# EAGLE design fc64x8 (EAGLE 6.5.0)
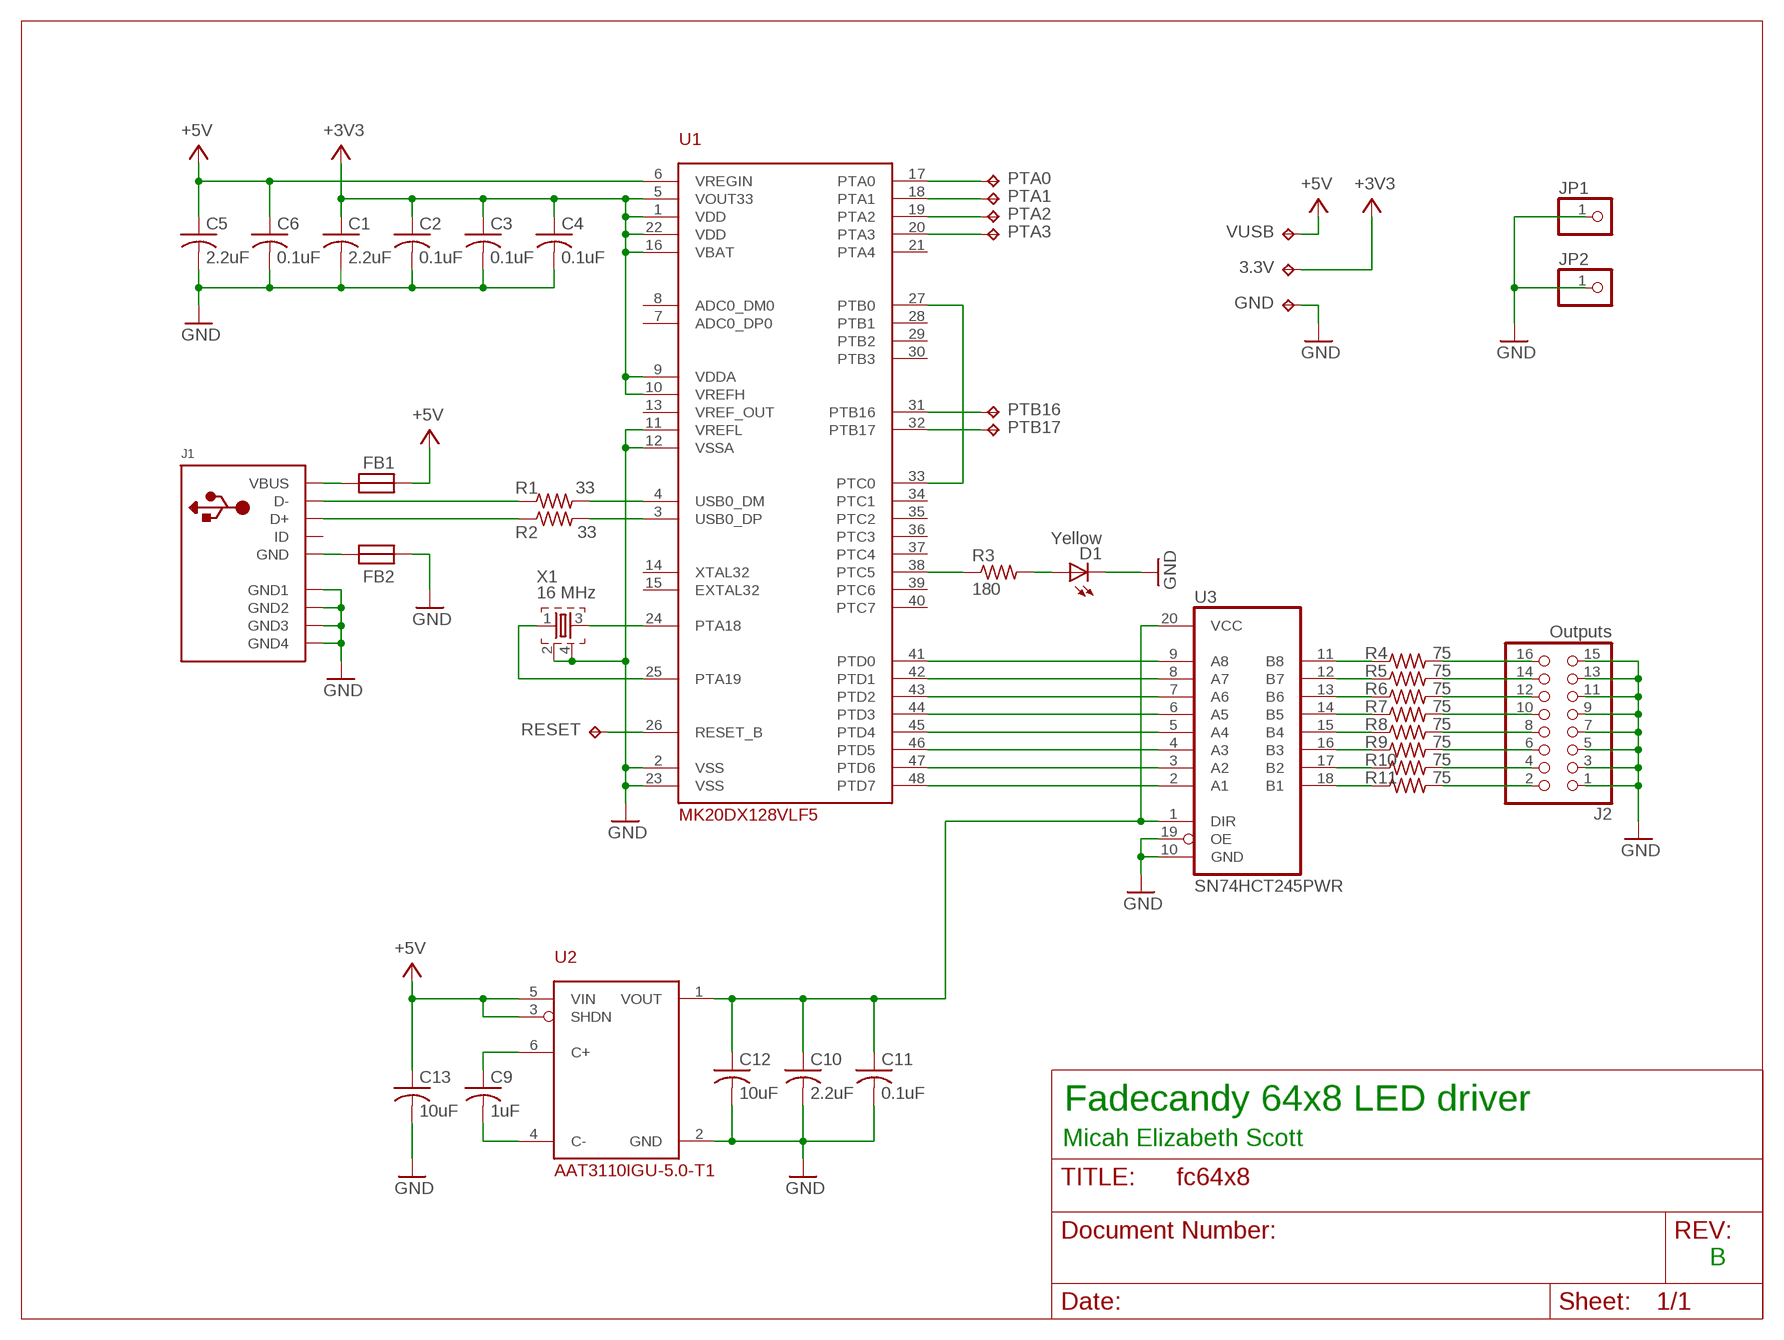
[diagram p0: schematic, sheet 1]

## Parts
3.3V  TPTP18SQ  [TP18SQ]
C1  2.2uF  C-US0805/NO-OUTLINE  [0805]
C2  0.1uF  C-US0805/NO-OUTLINE  [0805]
C3  0.1uF  C-US0805/NO-OUTLINE  [0805]
C4  0.1uF  C-US0805/NO-OUTLINE  [0805]
C5  2.2uF  C-US0805/NO-OUTLINE  [0805]
C6  0.1uF  C-US0805/NO-OUTLINE  [0805]
C9  1uF  C-US0805/NO-OUTLINE  [0805]
C10  2.2uF  C-US0805/NO-OUTLINE  [0805]
C11  0.1uF  C-US0805/NO-OUTLINE  [0805]
C12  10uF  C-US0805/NO-OUTLINE  [0805]
C13  10uF  C-US0805/NO-OUTLINE  [0805]
D1  Yellow  LEDCHIP-LED0805  [CHIP-LED0805]
FB1  FB0805/NO-OUTLINE  [0805]
FB2  FB0805/NO-OUTLINE  [0805]
GND  TPTP18SQ  [TP18SQ]
J1  USBMINIB  [USB-MINIB]
J2  Outputs  PINHD-2X8  [2X08]
JP1  PINHD-1X1  [1X01]
JP2  PINHD-1X1  [1X01]
PTA0  TPTP18SQ  [TP18SQ]
PTA1  TPTP18SQ  [TP18SQ]
PTA2  TPTP18SQ  [TP18SQ]
PTA3  TPTP18SQ  [TP18SQ]
PTB16  TPTP18SQ  [TP18SQ]
PTB17  TPTP18SQ  [TP18SQ]
R1  33  R-US_0805/NO-OUTLINE  [0805]
R2  33  R-US_0805/NO-OUTLINE  [0805]
R3  180  R-US_0805/NO-OUTLINE  [0805]
R4  75  R-US_0805/NO-OUTLINE  [0805]
R5  75  R-US_0805/NO-OUTLINE  [0805]
R6  75  R-US_0805/NO-OUTLINE  [0805]
R7  75  R-US_0805/NO-OUTLINE  [0805]
R8  75  R-US_0805/NO-OUTLINE  [0805]
R9  75  R-US_0805/NO-OUTLINE  [0805]
R10  75  R-US_0805/NO-OUTLINE  [0805]
R11  75  R-US_0805/NO-OUTLINE  [0805]
RESET  TPTP18SQ  [TP18SQ]
U1  MK20DX128VLF5  [LQFP48]
U2  AAT3110IGU-5.0-T1  AAT3110  [SOT23-6L]
U3  SN74HCT245PWR  74245PW  [TSSOP20]
VUSB  TPTP18SQ  [TP18SQ]
X1  16 MHz  TSX-32250  [TSX-3225]

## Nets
+3V3: 3.3V.TP C1.1 C2.1 C3.1 C4.1 U1.1(VDD) U1.5(VOUT33) U1.9(VDDA) U1.10(VREFH) U1.16(VBAT) U1.22(VDD)
+5V: C5.1 C6.1 C13.1 FB1.2 U1.6(VREGIN) U2.3(SHDN) U2.5(VIN) VUSB.TP
GND: C1.2 C2.2 C3.2 C4.2 C5.2 C6.2 C10.2 C11.2 C12.2 C13.2 D1.C FB2.2 GND.TP J1.GND1 J1.GND2 J1.GND3 J1.GND4 J2.1 J2.3 J2.5 J2.7 J2.9 J2.11 J2.13 J2.15 JP1.1 JP2.1 U1.2(VSS) U1.11(VREFL) U1.12(VSSA) U1.23(VSS) U2.2(GND) U3.10(GND) U3.19(OE) X1.2 X1.4
N$1: R3.1 U1.38(PTC5)
N$2: U1.24(PTA18) X1.3
N$3: D1.A R3.2
N$4: U1.25(PTA19) X1.1
N$5: FB1.1 J1.VBUS
N$6: U1.27(PTB0) U1.33(PTC0)
N$7: FB2.1 J1.GND
N$8: U1.41(PTD0) U3.9(A8)
N$9: J1.D- R1.1
N$10: J1.D+ R2.1
N$11: R1.2 U1.4(USB0_DM)
N$12: R2.2 U1.3(USB0_DP)
N$13: U1.42(PTD1) U3.8(A7)
N$14: U1.43(PTD2) U3.7(A6)
N$15: U1.44(PTD3) U3.6(A5)
N$16: U1.45(PTD4) U3.5(A4)
N$17: U1.46(PTD5) U3.4(A3)
N$18: U1.47(PTD6) U3.3(A2)
N$19: U1.48(PTD7) U3.2(A1)
N$20: R4.1 U3.11(B8)
N$21: C9.1 U2.6(C+)
N$22: C9.2 U2.4(C-)
N$23: R5.1 U3.12(B7)
N$24: R6.1 U3.13(B6)
N$25: R7.1 U3.14(B5)
N$26: R8.1 U3.15(B4)
N$27: C10.1 C11.1 C12.1 U2.1(VOUT) U3.1(DIR) U3.20(VCC)
N$28: R9.1 U3.16(B3)
N$29: R10.1 U3.17(B2)
N$30: R11.1 U3.18(B1)
N$31: J2.16 R4.2
N$32: J2.14 R5.2
N$33: J2.12 R6.2
N$34: J2.10 R7.2
N$35: J2.8 R8.2
N$36: J2.6 R9.2
N$37: J2.4 R10.2
N$38: J2.2 R11.2
N$39: RESET.TP U1.26(RESET_B)
N$40: PTA0.TP U1.17(PTA0)
N$41: PTA1.TP U1.18(PTA1)
N$42: PTA2.TP U1.19(PTA2)
N$43: PTA3.TP U1.20(PTA3)
N$45: PTB16.TP U1.31(PTB16)
N$46: PTB17.TP U1.32(PTB17)
Unconnected: J1.ID U1.7(ADC0_DP0) U1.8(ADC0_DM0) U1.13(VREF_OUT) U1.14(XTAL32) U1.15(EXTAL32) U1.21(PTA4) U1.28(PTB1) U1.29(PTB2) U1.30(PTB3) U1.34(PTC1) U1.35(PTC2) U1.36(PTC3) U1.37(PTC4) U1.39(PTC6) U1.40(PTC7)

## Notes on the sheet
- Fadecandy 64x8 LED driver
- Micah Elizabeth Scott
- B

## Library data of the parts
3.3V GND PTA0 PTA1-PTA3 PTB16 PTB17 RESET VUSB = testpad:TP: Test pad
C1-C6 C9-C13 = scanlime:C-US: CAPACITOR, American symbol
D1 = adafruit:LED: LED
FB1 FB2 = scanlime:FB
J1 = scanlime:USB: USB Connectors USBMINIB - Surface Mount Female Mini-B USB Connector 4UConnector: 06564 By microbuilder.eu Thru-hole RA Female Mini-B USB Connector 4UConnector: 18732 By ladyada.net
J2 = pinhead:PINHD-2X8: PIN HEADER
JP1 JP2 = pinhead:PINHD-1X1: PIN HEADER
R1-R11 = scanlime:R-US_: RESISTOR, American symbol
U1 = scanlime:MK20DX128VLF5: ARM Cortex-M4 microcontroller with USB. Freescale K20 series 50 MHz 16 K RAM 128 K Flash Lower pincount equivalent to Teensy 3.0 2013 Price: $2.66 qty 100 Digi-Key: MK20DX128VLF50-ND
U2 = scanlime:AAT3110: Switched capacitor boost converter
U3 = scanlime:74*245: Octal BUS TRANSCEIVER, 3-state
X1 = scanlime:TSX-3225: MHz RANGE CRYSTAL UNIT Source: Epson Toyocom

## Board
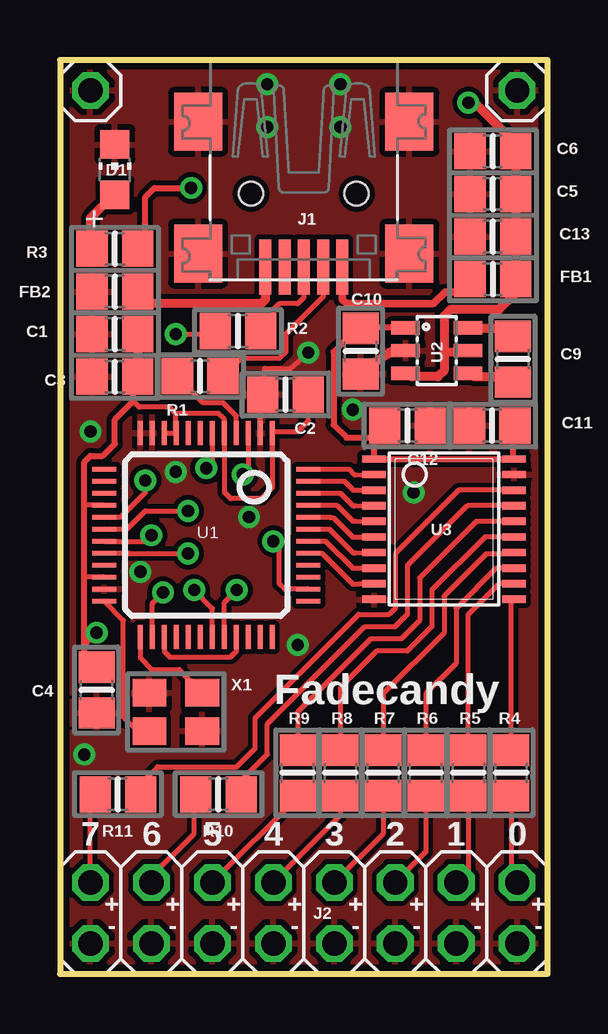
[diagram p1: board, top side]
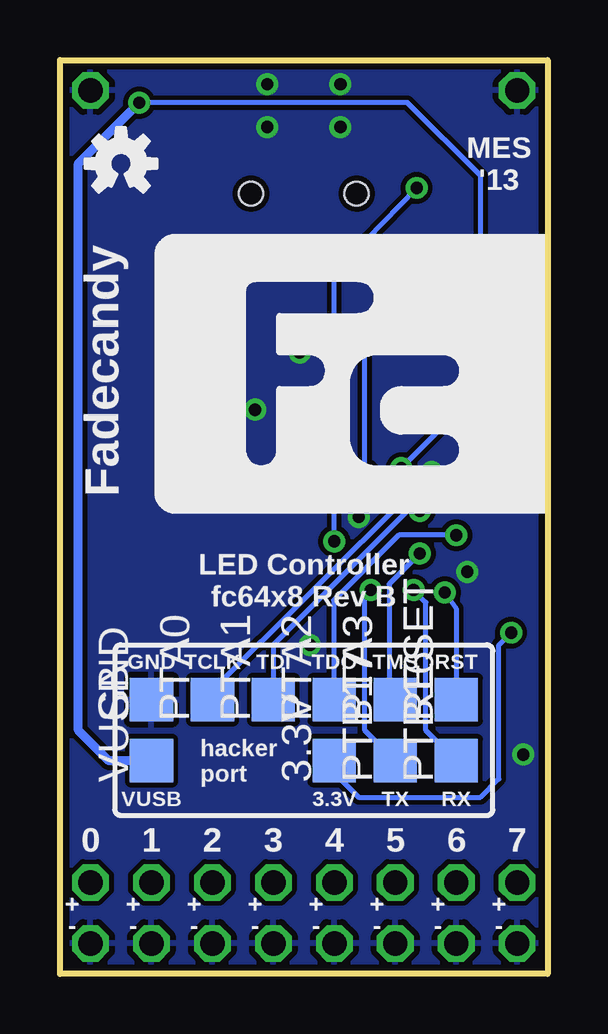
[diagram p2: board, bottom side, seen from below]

Size 20.32 x 38.1 mm. Coordinates in mm from the lower left corner, seen from the top.
Outline: 0,0 20.32,0 20.32,38.1 0,38.1 0,0
Copper layers (1*16): Top 0.035mm / dielectric 1.5mm / Bottom 0.035mm
Design rules "adafruit": minimum track width 8mil, minimum drill 15.5mil, track to track 8mil, track to pad 8mil, pad to pad 8mil, via to via 8mil, smd to smd 8mil, copper to edge 10mil, drill to drill 8mil, minimum pad ring 10mil, minimum via ring 8mil, stop-mask expansion 4mil, vias tented up to drill 20mil, thermal gap 10mil

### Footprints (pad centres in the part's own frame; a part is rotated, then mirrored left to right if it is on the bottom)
TP18SQ = smd 1.8 x 1.8: TP 0,0
0805 = smd 1.3 x 1.5: 1 -0.95,0; 2 0.95,0
CHIP-LED0805 = smd 1.2 x 1.2: A 0,-1.05; C 0,1.05
USB-MINIB = smd 0.5 x 2.308: D+ 0,4.064; D- -0.8,4.064; GND 1.6,4.064; ID 0.8,4.064; VBUS -1.6,4.064 | smd 2 x 2.4: GND1 -4.4,-2; GND2 -4.4,3.5; GND3 4.4,3.5; GND4 4.4,-2 | hole 1: -2.2,1; 2.2,1
2X08 = drill 1.016 octagon: 1 -8.89,-1.27; 2 -8.89,1.27; 3 -6.35,-1.27; 4 -6.35,1.27; 5 -3.81,-1.27; 6 -3.81,1.27; 7 -1.27,-1.27; 8 -1.27,1.27; 9 1.27,-1.27; 10 1.27,1.27; 11 3.81,-1.27; 12 3.81,1.27; 13 6.35,-1.27; 14 6.35,1.27; 15 8.89,-1.27; 16 8.89,1.27
1X01 = drill 1.016 octagon: 1 0,0
LQFP48 = smd 0.203 x 1: 1 -2.75,-4.25; 2 -2.25,-4.25; 3 -1.75,-4.25; 4 -1.25,-4.25; 5 -0.75,-4.25; 6 -0.25,-4.25; 7 0.25,-4.25; 8 0.75,-4.25; 9 1.25,-4.25; 10 1.75,-4.25; 11 2.25,-4.25; 12 2.75,-4.25; 25 2.75,4.25; 26 2.25,4.25; 27 1.75,4.25; 28 1.25,4.25; 29 0.75,4.25; 30 0.25,4.25; 31 -0.25,4.25; 32 -0.75,4.25; 33 -1.25,4.25; 34 -1.75,4.25; 35 -2.25,4.25; 36 -2.75,4.25 | smd 1 x 0.203: 13 4.25,-2.75; 14 4.25,-2.25; 15 4.25,-1.75; 16 4.25,-1.25; 17 4.25,-0.75; 18 4.25,-0.25; 19 4.25,0.25; 20 4.25,0.75; 21 4.25,1.25; 22 4.25,1.75; 23 4.25,2.25; 24 4.25,2.75; 37 -4.25,2.75; 38 -4.25,2.25; 39 -4.25,1.75; 40 -4.25,1.25; 41 -4.25,0.75; 42 -4.25,0.25; 43 -4.25,-0.25; 44 -4.25,-0.75; 45 -4.25,-1.25; 46 -4.25,-1.75; 47 -4.25,-2.25; 48 -4.25,-2.75
SOT23-6L = smd 0.55 x 1.2: 1 -0.95,-1.3; 2 0,-1.3; 3 0.95,-1.3; 4 0.95,1.3; 5 0,1.3; 6 -0.95,1.3
TSSOP20 = smd 0.305 x 0.991: 1 -2.925,-2.918; 2 -2.275,-2.918; 3 -1.625,-2.918; 4 -0.975,-2.918; 5 -0.325,-2.918; 6 0.325,-2.918; 7 0.975,-2.918; 8 1.625,-2.918; 9 2.275,-2.918; 10 2.925,-2.918; 11 2.925,2.918; 12 2.275,2.918; 13 1.625,2.918; 14 0.975,2.918; 15 0.325,2.918; 16 -0.325,2.918; 17 -0.975,2.918; 18 -1.625,2.918; 19 -2.275,2.918; 20 -2.925,2.918
TSX-3225 = smd 1.4 x 1.15: 1 -1.1,-0.8; 2 1.1,-0.8; 3 1.1,0.8; 4 -1.1,0.8

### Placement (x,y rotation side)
3.3V  8.89,8.89 90 bottom
C1  2.29,26.67 180 top
C2  9.4,24.16 180 top
C3  2.29,24.89 180 top
C4  1.52,11.84 270 top
C5  18.03,32.51 180 top
C6  18.03,34.29 180 top
C9  18.87,25.63 270 top
C10  12.52,25.96 270 top
C11  18.01,22.86 180 top
C12  14.48,22.86 0 top
C13  18.03,30.73 180 top
D1  2.29,33.53 0 top
FB1  18.03,28.96 0 top
FB2  2.29,28.45 180 top
GND  16.51,11.43 90 bottom
J1  10.16,33.53 180 top
J2  10.16,2.54 0 top
JP1  1.27,36.83 0 top
JP2  19.05,36.83 0 top
PTA0  13.97,11.43 90 bottom
PTA1  11.43,11.43 90 bottom
PTA2  8.89,11.43 90 bottom
PTA3  6.35,11.43 90 bottom
PTB16  3.81,8.89 90 bottom
PTB17  6.35,8.89 90 bottom
R1  5.84,24.92 180 top
R2  7.42,26.8 180 top
R3  2.29,30.23 180 top
R4  18.8,8.38 270 top
R5  17.02,8.38 270 top
R6  15.24,8.38 270 top
R7  13.46,8.38 270 top
R8  11.68,8.38 270 top
R9  9.91,8.38 270 top
R10  6.6,7.49 180 top
R11  2.41,7.49 180 top
RESET  3.81,11.43 90 bottom
U1  6.1,18.29 180 top
U2  15.7,25.98 270 top
U3  16,18.54 270 top
U$1  [OSHW-LOGO-S]  17.78,33.78 0 bottom
VUSB  16.51,8.89 90 bottom
X1  4.83,10.92 180 top

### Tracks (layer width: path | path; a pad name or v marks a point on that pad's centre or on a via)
+3V3  (via drill 0.51)
  Top 0.203: 1.02,16.51 1.04,16.54 U1.22 | 1.04,19.54 1.02,19.56 U1.16 | 1.02,13.46 1.02,13.72 v1.52,14.22 | U1.10 U1.9 | 1.02,12.95 C4.1 | U1.1 8.91,22.61 9.91,22.61 10.35,23.05 C2.1 | U1.9 4.83,22.56 4.83,23.37 | U1.1 8.89,22.58 | U1.9 4.83,22.52 | 8.85,21.8 U1.1 | 4.83,23.37 4.57,23.62 3.3,23.62 3.05,23.88 | U1.1 8.85,20.28 8.38,19.81 7.11,19.81 6.86,20.07 6.86,22.53 U1.5 6.85,23.13 6.6,23.37 4.83,23.37
  Top 0.254: 1.02,12.95 1.02,13.46 1.02,16.51 1.02,19.56 1.02,21.34 1.27,21.59 1.78,21.59 2.29,22.1 2.29,23.11 3.05,23.88 3.05,24.7 C3.1
  Top 0.381: C1.1 C3.1
  Bottom 0.203: 3.3V.TP 8.89,8.38 7.87,7.37 2.79,7.37 2.03,8.13 2.03,13.72 v1.52,14.22
+5V  (via drill 0.51)
  Top 0.203: 18.8,34.8 18.8,34.48 C6.1 | U1.6 6.35,21.33 v6.1,21.08
  Top 0.381: C6.1 C5.1 C13.1 FB1.2 18.98,28.38 18.29,27.69 16.26,27.69 16,27.43 16,25.91 | 16,25.91 16,25.15 15.75,24.89 14.67,24.89 U2.3 | U2.5 16.03,25.88 16,25.91 | v17.02,36.32 17.27,36.32 18.8,34.8
  Bottom 0.203: v6.1,21.08 2.79,24.38 2.79,33.27 5.84,36.32 v17.02,36.32
  Bottom 0.381: VUSB.TP 18.29,8.89 19.56,10.16 19.56,33.78 v17.02,36.32
GND  (via drill 0.51)
  Top 0.203: U1.2 8.35,24.03 C2.2 8.52,25.03 8.53,25.22 | 9.58,25.22 v10.34,25.91
  Top 0.254: 8.53,25.22 9.58,25.22
  Top 0.381: U2.2 13.89,25.98 13.01,25.43 12.86,25.3 C10.2
  other vias: 1.02,9.14 14.73,20.07 7.87,19.05 1.27,22.61 3.35,16.76 4.83,20.93 12.19,23.52 8.64,35.31 11.68,35.31 9.91,13.72 8.64,37.08 11.68,37.08
  pour Bottom: 0,38.1 20.32,38.1 20.32,0 0,0
  pour Top: 0,38.1 20.32,38.1 20.32,0 0,0
N$1  (via drill 0.51)
  Top 0.203: 3.56,30.55 R3.1 | U1.38 9.36,16.04 9.14,16.26 9.14,17.78 v8.89,18.03
  Top 0.254: 3.56,30.55 3.56,32.38 3.94,32.77 v5.46,32.77
  Bottom 0.203: v8.89,18.03 8.89,29.21 v5.46,32.77
N$2
  Top 0.203: X1.3 3.21,10.12 2.64,10.69 2.64,14.74 U1.24
N$3
  Top 0.381: D1.A 2.25,32.48 1.27,31.5 1.27,30.29 R3.2
N$4
  Top 0.203: U1.25 3.35,13.16 3.81,12.7 4.95,12.7 X1.1
N$5
  Top 0.305: J1.VBUS 11.76,28.12 11.94,27.94 15.56,27.94 16.05,28.42 16.94,28.42
  Top 0.381: 16.94,28.42 FB1.1
N$6
  Top 0.203: U1.27 4.35,13.43 4.57,13.21 7.11,13.21 7.35,13.44 U1.33
N$7
  Top 0.381: J1.GND 8.56,28.12 8.38,27.94 3.49,27.94 FB2.1
N$8
  Top 0.203: 12.45,16.26 U3.9 12.31,16.26 12.19,16.26 10.91,17.54 U1.41
N$9
  Top 0.203: J1.D- 10.96,28.23 9.4,26.67 9.4,25.91 9.14,25.65 7.53,25.65 R1.1
N$10
  Top 0.203: J1.D+ 10.16,28.19 9.91,27.94 9.14,27.94 8.89,27.69 8.89,27.32 R2.1
N$11
  Top 0.203: U1.4 7.35,23.26 6.81,23.8 5.96,23.8 R1.2
N$12  (via drill 0.51)
  Top 0.203: U1.3 7.85,21.05 v7.62,20.83 | v4.83,26.67 6.39,26.67 R2.2
  Bottom 0.203: v7.62,20.83 7.62,26.16 7.11,26.67 v4.83,26.67
N$13
  Top 0.203: 10.66,18.04 U1.42 11.07,18.03 12.19,16.92 12.32,16.92 U3.8
N$14
  Top 0.203: U1.43 10.66,18.54 10.92,18.54 11.23,18.54 12.22,17.55 12.31,17.55 U3.7
N$15
  Top 0.203: U1.44 11.26,19.04 11.28,19.02 11.38,19.02 12.19,18.21 12.32,18.21 U3.6
N$16
  Top 0.203: U1.45 11.53,19.54 12.19,18.87 12.32,18.87 U3.5
N$17
  Top 0.203: U1.46 11.69,20.04 12.22,19.51 12.31,19.51 U3.4
N$18
  Top 0.203: U1.47 11.85,20.54 12.22,20.17 12.32,20.17 U3.3
N$19
  Top 0.203: U1.48 12.03,21.04 12.27,20.8 12.31,20.8 U3.2
N$20
  Top 0.203: R4.1 18.8,15.49 U3.11
N$21
  Top 0.381: 18.75,26.5 C9.1 18.63,26.58 18.29,26.92 17.32,26.92 U2.6
N$22
  Top 0.381: 18.75,24.6 C9.2 18.5,24.68 18.29,24.89 17.27,24.89 U2.4
N$23
  Top 0.203: U3.12 18.3,16.27 17.02,14.99 R5.1
N$24
  Top 0.203: U3.13 18.19,16.92 16.51,15.24 16.51,12.95 15.24,11.68 R6.1
N$25
  Top 0.203: U3.14 18.88,17.53 17.78,17.53 16,15.75 16,14.22 13.46,11.68 R7.1
N$26
  Top 0.203: U3.15 17.71,18.22 15.49,16 15.49,14.48 14.48,13.46 13.21,13.46 11.68,11.94 R8.1
N$27
  Top 0.254: U2.1 12.84,26.93 12.95,26.42 12.74,26.42 | 12.74,26.42 C10.1 | 12.74,26.42 11.84,26.36 11.4,25.93 11.4,22.89 11.94,22.35 13.02,22.35 | 13.02,22.35 C12.1 | 13.02,22.35 13.08,22.29 U3.1 U3.20 18.88,21.5 18.88,22.79 C11.1
N$28
  Top 0.203: U3.16 17.34,18.87 14.99,16.51 14.99,14.73 14.22,13.97 12.95,13.97 9.91,10.92 R9.1
N$29
  Top 0.203: U3.17 16.98,19.52 14.48,17.02 14.48,14.99 13.97,14.48 12.7,14.48 8.64,10.41 8.64,9.14 7.55,8.06 R10.1
N$30
  Top 0.203: U3.18 16.61,20.17 13.97,17.53 13.97,15.24 13.72,14.99 12.45,14.99 8.13,10.67 8.13,9.4 7.37,8.64 4.06,8.64 3.36,7.93 R11.1
N$31
  Top 0.203: R4.2 18.8,4.06 J2.16
N$32
  Top 0.203: R5.2 17.02,4.32 J2.14
N$33
  Top 0.203: R6.2 15.24,5.08 J2.12
N$34
  Top 0.203: R7.2 13.46,5.84 J2.10
N$35
  Top 0.203: R8.2 11.68,6.6 J2.8
N$36
  Top 0.203: R9.2 9.91,7.37 J2.6
N$37
  Top 0.203: J2.4 3.81,4.06 5.59,5.84 5.59,7.43 R10.2
N$38
  Top 0.203: J2.2 1.27,7.3 R11.2
N$39  (via drill 0.51)
  Top 0.203: U1.26 3.85,15.45 v4.29,15.9
  Bottom 0.203: v4.29,15.9 3.81,15.24 RESET.TP
N$40  (via drill 0.51)
  Top 0.203: U1.17 2.53,19.04 3.56,20.07 v3.56,20.57
  Bottom 0.203: PTA0.TP 13.97,11.81 5.66,20.09 4.04,20.09 v3.56,20.57
N$41  (via drill 0.51)
  Top 0.203: U1.18 arc45 U1.18 2.79,18.54 3.56,19.3 v5.33,19.3
  Bottom 0.203: 11.18,12.19 11.43,12.19 PTA1.TP 11.43,13.72 5.84,19.3 v5.33,19.3
N$42  (via drill 0.51)
  Top 0.203: U1.19 arc45 U1.19 3.56,18.03 v3.81,18.29
  Bottom 0.203: v3.81,18.29 6.2,18.29 8.91,15.57 8.91,11.46 PTA2.TP
N$43  (via drill 0.51)
  Top 0.203: v5.33,17.53 2.64,17.53 2.88,17.54 U1.20
  Bottom 0.203: v5.33,17.53 6.6,16.26 6.6,11.68 PTA3.TP
N$45  (via drill 0.51)
  Top 0.203: U1.31 6.35,15.24 v5.59,16
  Bottom 0.203: PTB16.TP 5.08,10.16 5.08,15.49 v5.59,16
N$46  (via drill 0.51)
  Top 0.203: U1.32 6.85,15.48 v7.37,16
  Bottom 0.203: PTB17.TP 7.62,10.16 7.62,15.75 v7.37,16

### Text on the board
tPlace: Fadecandy | 7 | 6 | 5 | 4 | 3 | 2 | 1 | 0 | + | + | + | + | + | + | + | + | - | - | - | - | - | - | - | -
bPlace: MES / '13 | Fadecandy | LED Controller / fc64x8 Rev B | RST | TMS | TDO | TDI | TCLK | GND | hacker / port | RX | TX | 3.3V | VUSB | 7 | 6 | 5 | 4 | 3 | 2 | 1 | 0 | + | + | + | + | + | + | + | + | - | - | - | - | - | - | - | -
